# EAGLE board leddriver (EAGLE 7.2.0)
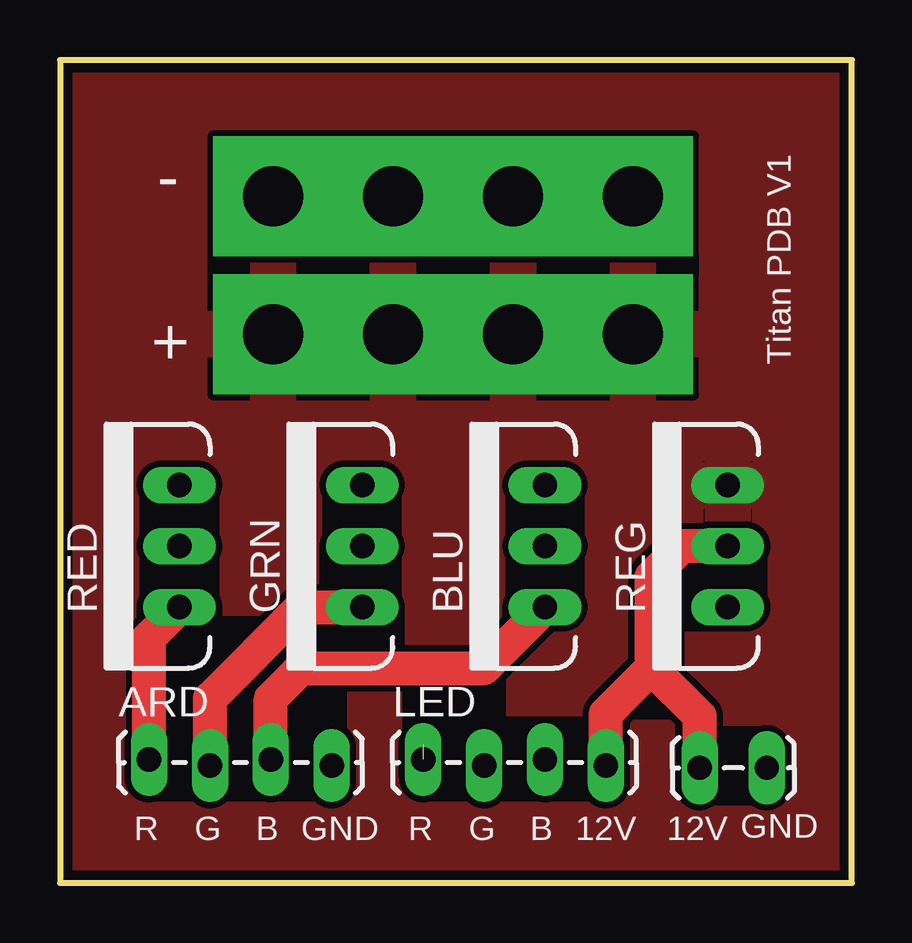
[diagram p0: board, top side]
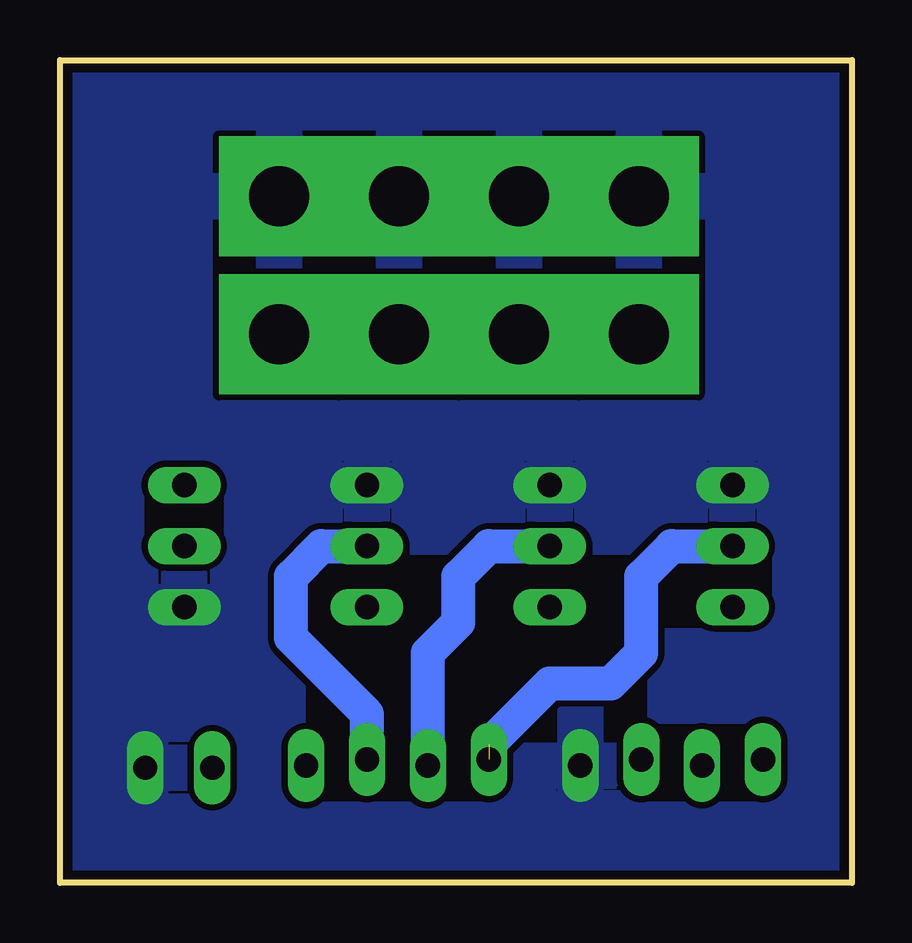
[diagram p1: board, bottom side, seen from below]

Size 33.02 x 34.29 mm. Coordinates in mm from the lower left corner, seen from the top.
Outline: 0,0 33.02,0 33.02,34.29 0,34.29 0,0
Copper layers (1*16): Top 0.0356mm / dielectric 1.5011mm / Bottom 0.0356mm
Design rules "oshpark": minimum track width 6mil, minimum drill 13mil, track to track 6mil, track to pad 6mil, pad to pad 6mil, via to via 6mil, smd to smd 6mil, copper to edge 15mil, drill to drill 6mil, minimum pad ring 7mil, minimum via ring 7mil, stop-mask expansion 3mil, vias tented up to drill 0mil, thermal gap 10mil

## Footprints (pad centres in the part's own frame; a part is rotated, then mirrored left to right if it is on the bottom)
1X02_LOCK_LONGPADS = drill 1.016 long: 1 -0.127,0; 2 2.667,0
1X04_LOCK_LONGPADS = drill 1.016 long: 1 0,0; 2 2.54,-0.254; 3 5.08,0; 4 7.62,-0.254
TO220V = drill 1.016 long: 1 -2.54,0; 2 0,0; 3 2.54,0
4WSP = drill 2.5 pad 5 square: P$1 0,0; P$2 5,0; P$3 10,0; P$4 15,0

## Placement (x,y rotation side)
12VOUT  [1X02_LOCK_LONGPADS]  26.8,4.8 0 top
ARD  [1X04_LOCK_LONGPADS]  3.71,5.14 0 top
BLU  MOSFET-PCHANNELFQP27P06  [TO220V]  20.22,14.04 90 top
GND  4WSP  [4WSP]  8.89,28.61 0 top
GRN  MOSFET-PCHANNELFQP27P06  [TO220V]  12.6,14.04 90 top
LED  [1X04_LOCK_LONGPADS]  15.14,5.14 0 top
RED  MOSFET-PCHANNELFQP27P06  [TO220V]  4.98,14.04 90 top
REG  MOSFET-PCHANNELFQP27P06  [TO220V]  27.84,14.04 90 top
VIN  4WSP  [4WSP]  8.89,22.86 0 top

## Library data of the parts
12VOUT ARD LED = SparkFun-Connectors
BLU GRN RED REG = User-Submitted
GND VIN = CYTLIB

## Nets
GND: 12VOUT.2 ARD.4 BLU.3 GND.P$1 GND.P$2 GND.P$3 GND.P$4 GRN.3 RED.3 REG.1
N$1: LED.1 RED.2
N$2: GRN.2 LED.2
N$3: BLU.2 LED.3
N$4: ARD.1 RED.1
N$5: ARD.2 GRN.1
N$6: ARD.3 BLU.1
N$7: 12VOUT.1 LED.4 REG.2
VIN: REG.3 VIN.P$1 VIN.P$2 VIN.P$3 VIN.P$4

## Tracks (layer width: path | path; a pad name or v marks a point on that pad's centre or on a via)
GND
  pour Bottom (isolate 0.254): 0,0 33.02,0 33.02,34.29 0,34.29
N$1  (1 unrouted)
  Bottom 1.422: 15.14,5.78 12.6,8.32 10.06,8.32 8.79,9.59 8.79,12.77 7.52,14.04 RED.2
N$2
  Bottom 1.422: LED.2 17.68,9.59 16.41,10.86 16.41,12.77 15.14,14.04 GRN.2
N$3
  Bottom 1.422: LED.3 20.22,7.05 23.39,10.22 23.39,12.77 22.12,14.04 BLU.2
N$4
  Top 1.422: ARD.1 3.71,10.22 RED.1
N$5
  Top 1.422: ARD.2 6.25,7.68 10.06,11.49 GRN.1
N$6
  Top 1.422: ARD.3 8.79,7.68 10.06,8.96 17.68,8.96 BLU.1
N$7
  Top 1.422: REG.2 25.93,14.04 24.66,12.77 24.66,8.96 | 24.66,8.96 26.67,6.95 12VOUT.1 | LED.4 22.76,7.05 24.66,8.96
VIN
  pour Top (isolate 0.254): 0,0 33.02,0 33.02,34.29 0,34.29

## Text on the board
tPlace: - | + | Titan PDB V1 | R | G | B | GND | R | G | B | 12V | 12V | GND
